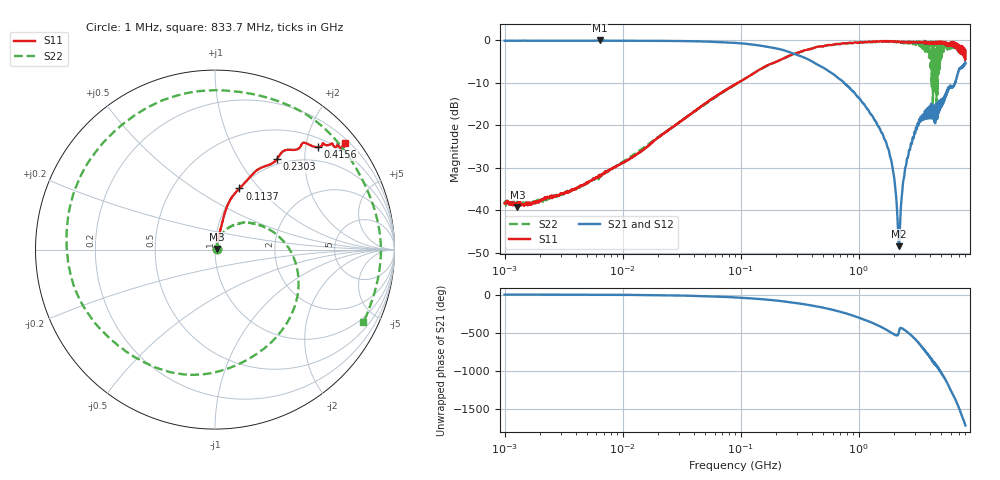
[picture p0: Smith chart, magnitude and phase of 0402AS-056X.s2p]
!s-Parameter Generated by FASTRON Sdn. Bhd.
!FASTRON P/N : 0402AS-056X
!Keysight Technologies: E5071C_MY46733604_B.14.02
!Date: Mon Dec 01 10:47:43 2025
!Version  :Rev00  Mon Dec 01 10:47:43 2025
!Data & Calibration Information:
!Freq  S11:SOLT2(ON)  S21:SOLT2(ON)  S12:SOLT2(ON)  S22:SOLT2(ON)
!PortZ  Port1:50+j0  Port2:50+j0
!When reading reference impedance value at option line is always used.
! Remarks : This data is being provided solely for informational purposes.
# Hz S dB R 50
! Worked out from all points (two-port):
!   1601 points, 1 MHz to 8 GHz, reference 50 ohm
!   highest |S21| = -0.04 dB at 6.4 MHz (marker M1); lowest = -48.4 dB at 2.189 GHz (marker M2)
!   |S21| within 3 dB of the highest: start of sweep to 274.2 MHz
!   lowest |S11| = -39.2 dB at 1.284 MHz (marker M3), VSWR 1.02, Z = 51 + j0.432 ohm
!   |S11| at or under -10 dB: start of sweep to 94.7 MHz
!   |S22| runs from -38.9 to -0.1 dB; largest |S21 - S12| = 0.014
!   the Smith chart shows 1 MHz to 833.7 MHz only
!   S11 on the Smith chart (normalised r, x): 1 MHz: 1.02, +0.01; 113.7 MHz: 1.00, +0.79; 230.3 MHz: 0.92, +1.48; 415.6 MHz: 0.68, +2.25; 833.7 MHz: 0.29, +2.77
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1000000  -38.30 20.7  -0.11 -0.4  -0.10 -0.5  -37.90 20.1
1283835  -39.20 22.7  -0.14 -0.6  -0.11 -0.5  -37.80 24.6
4479405  -34.20 55.0  -0.12 -2.0  -0.10 -2.0  -34.20 54.5
6400096  -31.60 61.5  -0.04 -2.8  -0.02 -2.7  -31.70 56.7
2.00676e7  -22.80 74.3  -0.14 -8.8  -0.14 -8.7  -22.70 67.9
8.994653e7  -10.40 72.3  -0.62 -37.8  -0.61 -37.7  -10.40 24.8
1.136953e8  -8.71 68.2  -0.86 -47.2  -0.86 -47.2  -8.69 10.6
2.303365e8  -4.27 55.6  -2.33 -90.1  -2.32 -90.0  -4.33 -60.2
4.006501e8  -2.00 46.4  -4.95 -145.0  -4.94 -145.0  -1.92 -159.0
4.15608e8  -1.84 44.8  -5.21 -149.0  -5.20 -149.0  -1.80 -166.0
6.141436e8  -1.01 40.3  -8.01 155.0  -8.00 155.0  -1.03 88.0
8.33667e8  -0.57 39.3  -11.20 97.9  -11.20 97.7  -0.71 -26.1
1.1258e9  -0.34 42.7  -15.30 27.2  -15.30 27.1  -0.54 -173.0
1.334081e9  -0.27 48.5  -18.30 -19.9  -18.30 -20.0  -0.41 86.5
1.542898e9  -0.26 55.0  -21.50 -65.4  -21.50 -65.4  -0.27 -11.8
1.7949e9  -0.21 61.9  -25.80 -121.0  -25.90 -121.0  -0.38 -134.0
2.189041e9  -0.29 70.3  -48.40 -126.0  -48.30 -127.0  -0.59 29.1
2.618947e9  -0.46 81.3  -27.30 -141.0  -27.30 -141.0  -0.33 -176.0
2.985754e9  -0.41 91.8  -21.80 136.0  -21.70 136.0  -0.68 0.6
3.345355e9  -0.48 101.0  -18.00 49.7  -17.90 49.4  -1.51 -176.0
3.710194e9  -0.69 110.0  -17.30 -28.8  -17.30 -29.1  -0.27 20.0
8e9  -2.42 -113.0  -5.42 81.0  -5.42 80.8  -4.19 119.0
